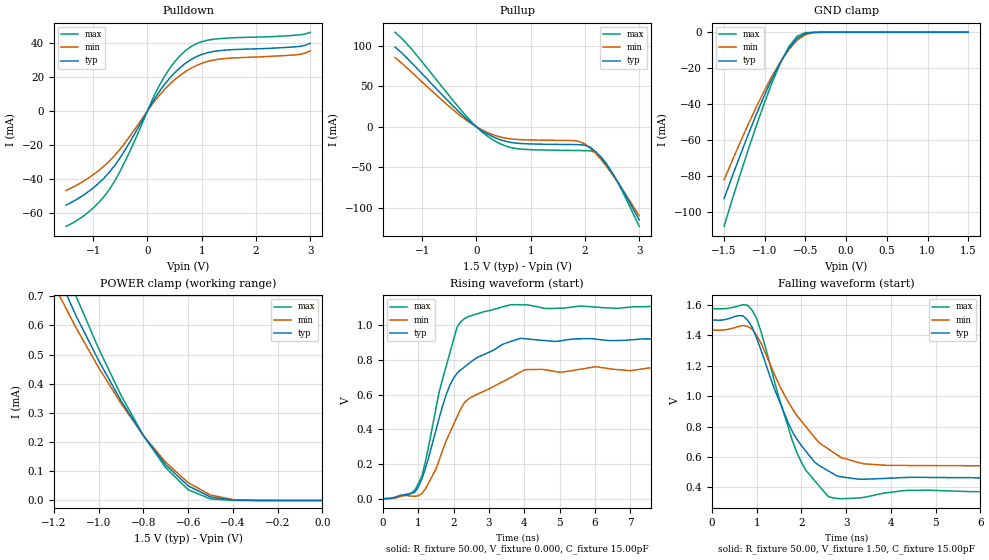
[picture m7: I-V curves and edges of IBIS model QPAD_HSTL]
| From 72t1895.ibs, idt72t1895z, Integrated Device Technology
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|   Model QPAD_HSTL
[Model]   QPAD_HSTL
Model_type   3-state
Polarity   Non-Inverting
Enable   Active-High
Vmeas =  0.750V
C_comp   3.00pF   NA   NA
[Temperature Range]   25.00   85.00   -40.00
[Voltage Range]   1.50V   1.40V   1.60V
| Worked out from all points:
|   slope of the pulldown table from 0 to 0.225 V, typ, clamps not added: 19.3 ohm
|   slope of the pullup table from 0 to 0.225 V, typ, clamps not added: 23.5 ohm
|   GND clamp passes 1 mA (typ) near -0.51 V on its own axis
|   POWER clamp passes 1 mA (typ) near -1.28 V on its own axis
|   rising waveform, R_fixture 50.00, V_fixture 0.000, C_fixture 15.00pF: 20-80 % time 932ps typ, 1.22ns min, 742ps max; typ from 0 V to 0.916 V
|   falling waveform, R_fixture 50.00, V_fixture 1.50, C_fixture 15.00pF: 20-80 % time 904ps typ, 1.08ns min, 740ps max; typ from 1.5 V to 0.463 V
[Pulldown]
| voltage   I(typ)   I(min)   I(max)
-1.5V     -55.54mA   -46.94mA   -68mA
-1.1V     -47.85mA   -39.79mA   -60mA
-900mV    -42.65mA   -35.17mA   -54.12mA
-700mV    -36.05mA   -29.51mA   -46.23mA
-400mV    -22.33mA   -18.22mA   -28.88mA
200mV     10.57mA    8.525mA    13.92mA
400mV     19.01mA    15.49mA    24.67mA
700mV     28.12mA    23.26mA    35.58mA
900mV     32.02mA    26.81mA    39.69mA
1.2V      35.04mA    29.92mA    42.26mA
2.7V      37.81mA    33.05mA    44.66mA
3V        39.96mA    35.49mA    46.45mA
[Pullup]
| voltage   I(typ)   I(min)   I(max)
-1.5V     98.65mA    85.66mA    117mA
-1.2V     79.68mA    67.92mA    96.54mA
-300mV    17.26mA    14.08mA    22.02mA
0V        0A         0A         10pA
300mV     -12.12mA   -9.575mA   -15.95mA
800mV     -20.5mA    -15.79mA   -27.4mA
1.9V      -22.02mA   -18.14mA   -29.27mA
2.1V      -25.42mA   -26.39mA   -29.62mA
2.2V      -30.83mA   -32.98mA   -31.59mA
2.3V      -38.24mA   -40.65mA   -37.27mA
2.5V      -56.93mA   -58.35mA   -56.49mA
3V        -115mA     -110mA     -123mA
[GND_clamp]
| voltage   I(typ)   I(min)   I(max)
-1.5V     -92.56mA   -82.16mA   -108mA
-1.4V     -80.26mA   -71.45mA   -93.09mA
-1.2V     -56.53mA   -50.9mA    -64.94mA
-1.1V     -45.3mA    -41.22mA   -51.5mA
-1V       -34.68mA   -32.07mA   -38.72mA
-900mV    -24.85mA   -23.59mA   -26.87mA
-800mV    -16.08mA   -15.96mA   -16.35mA
-700mV    -8.721mA   -9.411mA   -7.76mA
-600mV    -3.357mA   -4.326mA   -2.135mA
-500mV    -667uA     -1.241mA   -218uA
-400mV    -58.99uA   -179uA     -9.374uA
1.5V      15.04nA    17.39nA    15nA
[POWER_clamp]
| voltage   I(typ)   I(min)   I(max)
-1.5V     2.847mA    1.929mA    4.371mA
-1.2V     803uA      739uA      910uA
-1.1V     632uA      591uA      699uA
-1V       480uA      456uA      521uA
-900mV    342uA      333uA      361uA
-800mV    222uA      223uA      223uA
-700mV    122uA      131uA      112uA
-600mV    50.34uA    61.26uA    37.18uA
-500mV    11.87uA    18.7uA     5.404uA
-400mV    1.358uA    3.086uA    373nA
0V        15.04nA    15.59nA    16nA
[Ramp]
| variable   typ   min   max
dV/dt_r   0.55/0.49n   0.45/0.62n   0.67/0.40n
dV/dt_f   0.63/0.63n   0.55/0.73n   0.73/0.50n
R_load = 50.00
[Rising Waveform]
R_fixture = 50.00
V_fixture = 0.000
C_fixture = 15.00pF
R_dut = 0.75
L_dut = 8.10nH
C_dut = 0.53pF
| time   V(typ)   V(min)   V(max)
0s        0V         0V         0V
800ps     29.96mV    15.26mV    32.19mV
1.1ns     112mV      29.69mV    127mV
1.5ns     393mV      170mV      519mV
1.8ns     604mV      338mV      770mV
2.1ns     723mV      472mV      989mV
2.4ns     774mV      572mV      1.049V
3.4ns     891mV      675mV      1.107V
4.1ns     921mV      745mV      1.118V
9.9ns     916mV      753mV      1.102V
[Falling Waveform]
R_fixture = 50.00
V_fixture = 1.50
C_fixture = 15.00pF
R_dut = 0.75
L_dut = 8.10nH
C_dut = 0.53pF
| time   V(typ)   V(min)   V(max)
0s        1.5V       1.433V     1.575V
700ps     1.527V     1.464V     1.601V
900ps     1.453V     1.44V      1.564V
1.1ns     1.3V       1.347V     1.422V
1.4ns     1.045V     1.142V     1.094V
1.9ns     716mV      872mV      628mV
2.1ns     638mV      799mV      512mV
2.6ns     509mV      653mV      340mV
3.9ns     460mV      545mV      365mV
9.9ns     463mV      542mV      373mV
